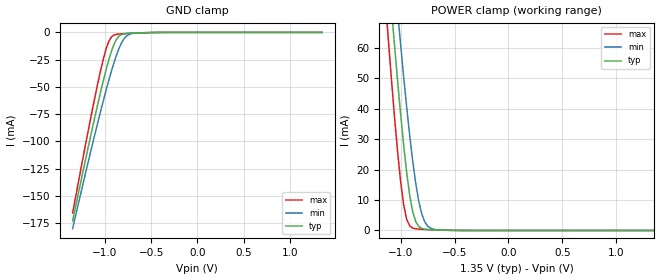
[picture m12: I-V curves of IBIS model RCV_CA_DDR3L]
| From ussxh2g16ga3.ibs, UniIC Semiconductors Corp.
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|   Model RCV_CA_DDR3L
[Model] RCV_CA_DDR3L
Model_type Input
Vinl =  0.540V
Vinh =  0.810V
C_comp   0.690pF   0.690pF   0.690pF
[Model Spec]
Vinh   0.810V   0.776V   0.860V
Vinl   0.540V   0.506V   0.590V
[Temperature Range]   25.000   95.000   -40.000
[Voltage Range]   1.350V   1.283V   1.450V
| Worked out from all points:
|   GND clamp passes 1 mA (typ) near -0.77 V on its own axis
|   POWER clamp passes 1 mA (typ) near -0.82 V on its own axis
[GND_clamp]
|Voltage   I(typ)   I(min)   I(max)
-1.35V    -172.8mA   -179.9mA   -165.6mA
-1.126V   -83.84mA   -99.28mA   -66.45mA
-1.042V   -52.75mA   -70.63mA   -32.99mA
-986mV    -33.67mA   -52.44mA   -14.65mA
-958mV    -25.01mA   -43.77mA   -8.113mA
-930mV    -17.28mA   -35.47mA   -4.15mA
-874mV    -6.141mA   -20.55mA   -1.759mA
-818mV    -1.856mA   -9.196mA   -1.325mA
-762mV    -946uA     -3.027mA   -1.066mA
-678mV    -590.6uA   -657uA     -726.8uA
-510mV    -182.2uA   -145.1uA   -204.8uA
1.35V     0A         0A         0A
[POWER_clamp]
|Voltage   I(typ)   I(min)   I(max)
-1.35V    193.8mA    208.2mA    178.6mA
-1.142V   97mA       117.7mA    74.79mA
-1.114V   84.56mA    105.9mA    61.67mA
-1.086V   72.37mA    94.37mA    48.99mA
-1.058V   60.5mA     82.99mA    36.93mA
-1.03V    49.05mA    71.85mA    25.78mA
-1.002V   38.16mA    61.01mA    16.03mA
-946mV    19.06mA    40.6mA     3.668mA
-890mV    6.184mA    22.84mA    784uA
-806mV    668.8uA    5.465mA    387.6uA
-694mV    183.7uA    385.9uA    217.7uA
1.35V     0A         0A         0A
